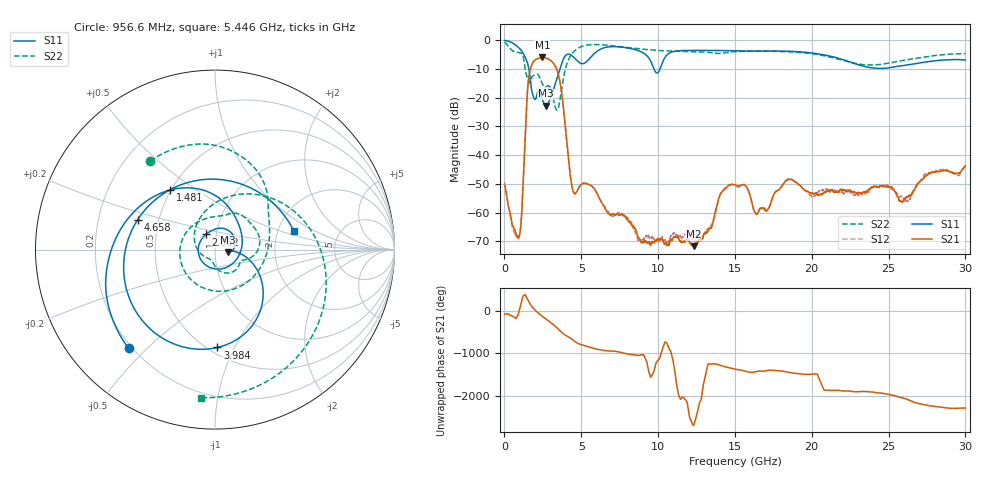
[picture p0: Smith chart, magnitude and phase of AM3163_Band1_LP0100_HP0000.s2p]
!Agilent Technologies,E8364B,MY43040894,A.07.50.67
!Agilent E8364B: A.07.50.67
!Date: Thursday, August 20, 2020 11:26:26
!Correction: S11(Full 2 Port(1,2))
!S21(Full 2 Port(1,2))
!S12(Full 2 Port(1,2))
!S22(Full 2 Port(1,2))
!S2P File: Measurements: S11, S21, S12, S22:
# Hz S  dB  R 50
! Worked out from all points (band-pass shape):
!   3201 points, 10 MHz to 30 GHz, reference 50 ohm
!   highest |S21| = -5.99 dB at 2.465 GHz (marker M1); lowest = -71.7 dB at 12.32 GHz (marker M2)
!   |S21| within 3 dB of the highest: 1.749 GHz to 3.307 GHz (1.558 GHz wide, 61.6 % of centre)
!   lowest |S11| = -22.8 dB at 2.7 GHz (marker M3), VSWR 1.16, Z = 57.6 - j1.61 ohm
!   |S11| at or under -10 dB: 1.587 GHz to 3.608 GHz (2.02 GHz wide, 77.8 % of centre); 9.733 GHz to 10.12 GHz (388.4 MHz wide, 3.91 % of centre)
!   |S22| runs from -24.3 to -0.6 dB; largest |S21 - S12| = 0.0095
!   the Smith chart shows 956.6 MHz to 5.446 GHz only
!   S11 on the Smith chart (normalised r, x): 956.6 MHz: 0.19, -0.44; 1.481 GHz: 0.50, +0.40; 2.062 GHz: 0.89, +0.15; 3.984 GHz: 0.55, -0.86; 4.658 GHz: 0.38, +0.16; 5.446 GHz: 2.45, +0.64
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1e7  -0.06 -9.0  -50.47 -73.6  -49.45 165.3  -0.64 -26.4
4.973375e8  -0.86 -66.2  -63.83 -116.8  -64.71 -165.0  -3.49 -149.4
9.565594e8  -2.72 -131.2  -68.31 1.9  -68.16 171.1  -4.27 126.3
1.481384e9  -7.63 126.8  -18.94 -63.7  -18.90 -63.6  -12.81 -94.8
2.062441e9  -20.12 120.9  -6.62 -1.0  -6.62 -1.0  -11.95 26.9
2.465431e9  -20.57 -5.3  -5.99 -122.4  -6.00 -122.5  -15.17 -19.3
2.699728e9  -22.78 -11.0  -6.19 173.3  -6.20 173.3  -16.14 -27.0
3.243297e9  -16.22 -10.4  -8.43 21.4  -8.44 21.4  -22.05 -95.2
3.983675e9  -5.26 -88.6  -31.34 145.6  -31.32 146.2  -9.64 68.3
4.65845e9  -6.70 158.9  -53.05 -18.9  -53.08 -20.1  -3.25 -29.2
5.014581e9  -8.11 92.8  -50.10 -75.0  -50.20 -75.5  -2.20 -62.3
5.445688e9  -6.90 13.2  -50.05 -122.2  -50.10 -123.0  -1.63 -95.4
6.345388e9  -2.87 -93.4  -56.58 155.1  -56.71 156.9  -1.57 -149.5
7.441897e9  -2.28 -169.6  -60.97 113.7  -60.10 117.0  -2.17 159.0
8.772703e9  -3.72 119.9  -69.07 35.0  -69.49 44.1  -2.97 105.5
1.000979e10  -11.13 100.2  -69.27 -80.4  -69.75 32.2  -3.53 59.6
1.232464e10  -3.53 10.3  -71.69 -163.7  -69.28 134.0  -3.95 -19.7
1.5005e10  -3.63 -72.2  -50.35 66.2  -50.50 66.9  -3.95 -90.5
2.000958e10  -4.42 163.4  -53.28 -51.4  -54.53 -55.8  -4.69 136.4
2.275554e10  -8.03 60.2  -52.63 -104.5  -53.97 -98.5  -7.98 21.2
2.500479e10  -9.61 -62.0  -51.08 -168.5  -50.92 -170.1  -7.97 -92.5
3e10  -6.90 104.9  -43.68 -136.0  -43.58 -129.4  -4.62 102.3
